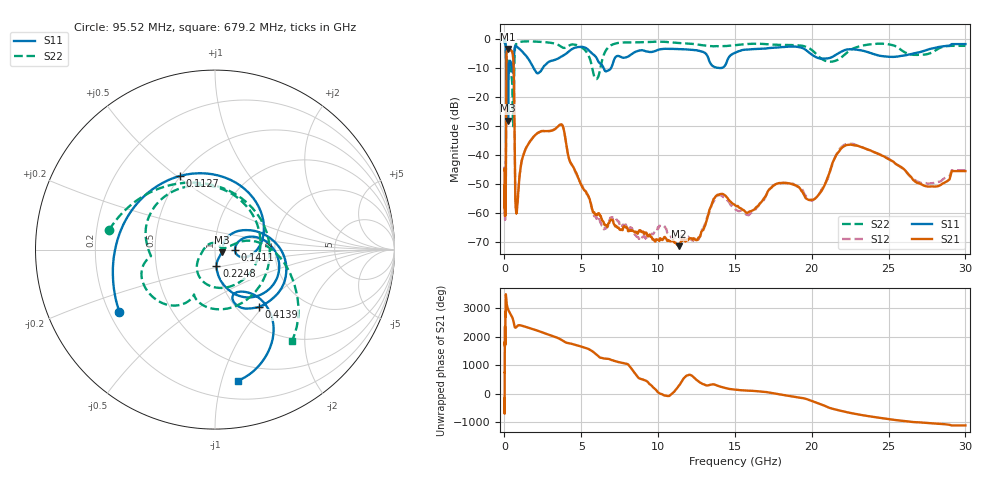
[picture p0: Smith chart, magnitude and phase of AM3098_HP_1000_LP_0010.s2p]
! Date/Time: Thu, Feb 28, 2019 8:39 AM
! Network Analyzer: Agilent Technologies E8364B Rev: A.07.50.67
! Sweep from 0.010 to 30.000 GHz, 1601 Points, Sweep Type: LOG
! Power Supply: 5.023 V, 0.002 A
# Hz S DB R 50
!freq MagS11 AngS11 MagS21 AngS21 MagS12 AngS12 MagS22 AngS22
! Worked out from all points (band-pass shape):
!   1601 points, 10 MHz to 30 GHz, reference 50 ohm
!   highest |S21| = -3.31 dB at 236.3 MHz (marker M1); lowest = -71.4 dB at 11.36 GHz (marker M2)
!   |S21| within 3 dB of the highest: 127.3 MHz to 566.2 MHz (438.9 MHz wide, 127 % of centre)
!   lowest |S11| = -28.1 dB at 236.3 MHz (marker M3), VSWR 1.08, Z = 53.8 - j1.63 ohm
!   |S11| at or under -10 dB: 198.2 MHz to 289.5 MHz (91.22 MHz wide, 37.4 % of centre); 1.909 GHz to 2.475 GHz (565.4 MHz wide, 25.8 % of centre); 6.47 GHz to 6.923 GHz (452.5 MHz wide, 6.76 % of centre)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
!   |S22| runs from -30.0 to -0.6 dB; largest |S21 - S12| = 0.011
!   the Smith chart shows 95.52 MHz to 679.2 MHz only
!   S11 on the Smith chart (normalised r, x): 95.52 MHz: 0.24, -0.28; 112.7 MHz: 0.50, +0.52; 141.1 MHz: 1.25, -0.01; 224.8 MHz: 1.00, -0.18; 413.9 MHz: 1.24, -0.95; 679.2 MHz: 0.35, -1.13
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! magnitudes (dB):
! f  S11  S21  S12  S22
! 10 MHz  -0.3  -45.2  -45.9  -0.6
! 38.04 MHz  -0.5  -61.1  -59.8  -0.8
! 95.52 MHz  -3.9  -41.6  -42.0  -4.4
! 112.7 MHz  -6.9  -16.4  -16.4  -10.3
! 141.1 MHz  -19.1  -4.5  -4.4  -11.0
! 144.7 MHz  -18.4  -4.3  -4.3  -10.5
! 184 MHz  -8.5  -3.9  -3.9  -7.1
! 224.8 MHz  -20.8  -3.4  -3.3  -8.8
! 236.3 MHz  -28.1  -3.3  -3.3  -8.9
! 413.9 MHz  -7.9  -3.7  -3.7  -11.3
! 550.5 MHz  -11.5  -5.6  -5.5  -28.4
! 617.6 MHz  -6.2  -13.5  -13.4  -13.7
! 679.2 MHz  -2.6  -44.3  -44.3  -3.5
! 781.4 MHz  -2.4  -59.9  -58.2  -1.4
! 2.084 GHz  -11.5  -32.7  -32.6  -0.7
! 3.723 GHz  -5.9  -29.4  -29.4  -2.6
! 5.989 GHz  -6.3  -60.4  -62.0  -13.7
! 7.926 GHz  -6.2  -64.9  -64.4  -1.0
! 11.36 GHz  -3.3  -71.4  -68.6  -1.2
! 20.2 GHz  -5.9  -55.1  -55.0  -4.6
! 22.56 GHz  -3.4  -36.4  -36.1  -3.5
! 30 GHz  -1.6  -45.5  -45.2  -2.2
